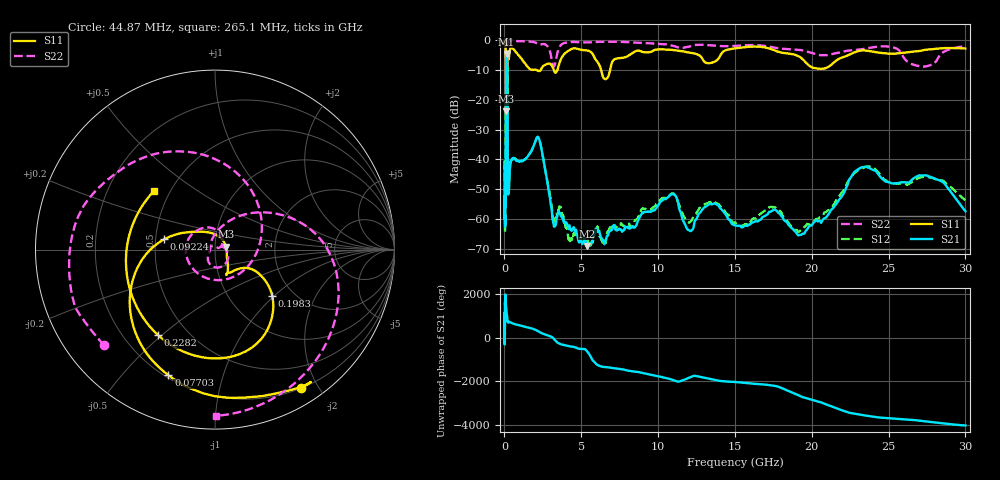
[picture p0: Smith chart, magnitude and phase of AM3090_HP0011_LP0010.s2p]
! Date/Time: Thu, Feb 28, 2019 1:56 PM
! Network Analyzer: Agilent Technologies E8364B Rev: A.07.50.67
! Sweep from 0.010 to 30.000 GHz, 1601 Points, Sweep Type: LOG
! Power Supply: 5.023 V, 0.002 A
# Hz S DB R 50
!freq MagS11 AngS11 MagS21 AngS21 MagS12 AngS12 MagS22 AngS22
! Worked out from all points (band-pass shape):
!   1601 points, 10 MHz to 30 GHz, reference 50 ohm
!   highest |S21| = -4.67 dB at 139.7 MHz (marker M1); lowest = -69.0 dB at 5.392 GHz (marker M2)
!   |S21| within 3 dB of the highest: 101.4 MHz to 184.2 MHz (82.74 MHz wide, 57.9 % of centre)
!   lowest |S11| = -24.0 dB at 100.4 MHz (marker M3), VSWR 1.14, Z = 56.5 + j1.92 ohm
!   |S11| at or under -10 dB: 2.055 GHz to 2.361 GHz (306.2 MHz wide, 13.9 % of centre); 3.205 GHz to 3.448 GHz (242.8 MHz wide, 7.3 % of centre); 6.288 GHz to 6.877 GHz (589 MHz wide, 8.95 % of centre)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
!   |S22| runs from -35.2 to -0.2 dB; largest |S21 - S12| = 0.015
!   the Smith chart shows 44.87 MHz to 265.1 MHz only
!   S11 on the Smith chart (normalised r, x): 44.87 MHz: 0.20, -1.78; 77.03 MHz: 0.21, -0.67; 92.24 MHz: 0.56, +0.07; 198.3 MHz: 1.57, -0.98; 228.2 MHz: 0.34, -0.48; 265.1 MHz: 0.41, +0.34
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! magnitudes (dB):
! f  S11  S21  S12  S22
! 10 MHz  -0.2  -43.0  -40.3  -0.5
! 38.04 MHz  -0.5  -58.8  -64.1  -1.3
! 44.87 MHz  -0.8  -55.0  -55.4  -1.7
! 77.03 MHz  -2.5  -46.6  -47.3  -5.0
! 92.24 MHz  -10.8  -15.5  -15.5  -15.3
! 100.4 MHz  -24.0  -8.1  -8.0  -16.1
! 127.7 MHz  -16.4  -4.8  -4.8  -35.2
! 139.7 MHz  -16.4  -4.7  -4.7  -25.2
! 144.7 MHz  -16.3  -4.7  -4.7  -22.1
! 177.7 MHz  -14.2  -6.5  -6.5  -31.2
! 198.3 MHz  -7.7  -16.2  -16.1  -10.6
! 228.2 MHz  -4.9  -50.7  -49.6  -1.6
! 265.1 MHz  -6.5  -51.0  -51.0  -0.7
! 550.5 MHz  -3.0  -39.7  -39.9  -0.3
! 2.084 GHz  -10.1  -33.0  -33.0  -1.0
! 3.236 GHz  -10.4  -62.6  -60.2  -8.8
! 5.392 GHz  -3.5  -69.0  -67.1  -0.8
! 7.926 GHz  -5.6  -62.7  -61.7  -0.7
! 10.81 GHz  -3.3  -52.0  -51.7  -1.8
! 19.41 GHz  -6.5  -64.9  -63.3  -3.5
! 23.48 GHz  -3.5  -42.5  -42.5  -2.9
! 30 GHz  -2.9  -57.4  -53.7  -2.2
